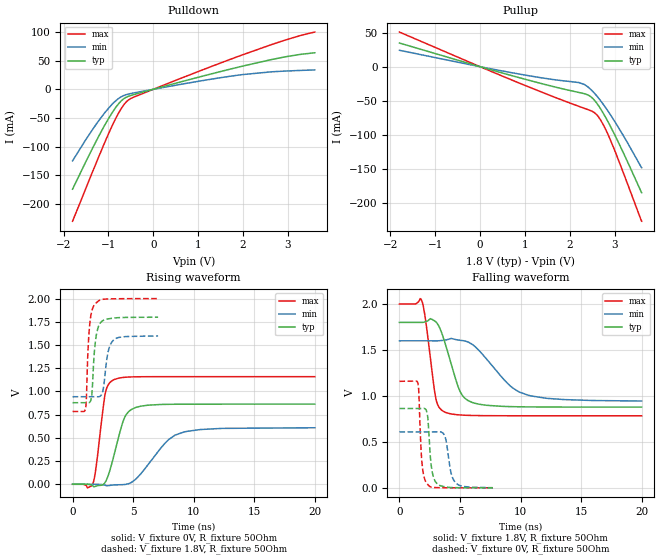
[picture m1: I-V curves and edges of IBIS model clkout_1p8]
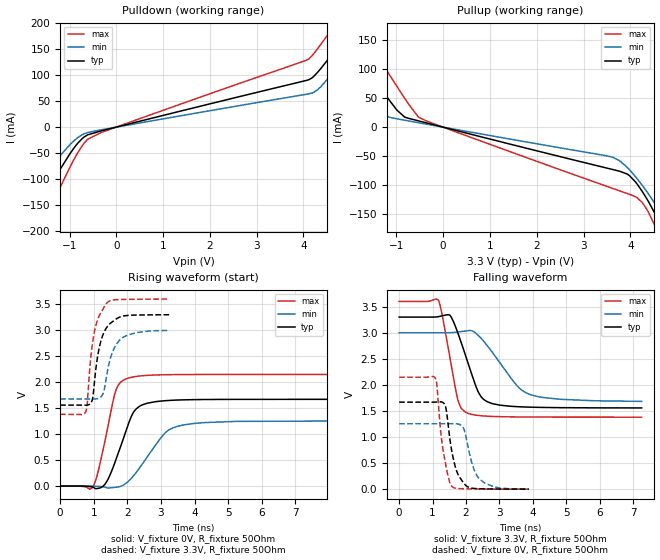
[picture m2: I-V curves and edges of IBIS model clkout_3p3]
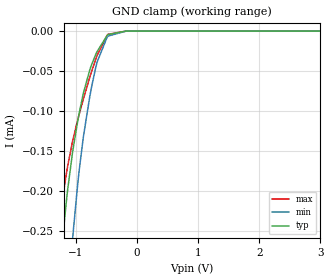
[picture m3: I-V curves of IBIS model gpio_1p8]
|Texas Instruments Incorporated
| TPS657095 Embedded Camera Module PMIC
| Marketing part#   Digital Voltage Range   Package-type   #pins
| TPS657095YFFR   3.7V-6V   DSBGA   16
| TPS657095YFFT   3.7V-6V   DSBGA   16
[IBIS Ver]   4.1
[File name]   tps657095.ibs
[File Rev]   1.0
[Date]   9/18/2015
[Source]
| Texas Instruments Incorporated.
| Analog-eLab Design Center, HPA
| 12500 TI Blvd
| Dallas, TX -75243
[Notes]   Revision History:
| Rev 1.0: 9/18/2015
| - Initial version of the model
| - Model generated from simulations in SPECTRE
| - Model matched to SPECTRE simulation
| - C_comp although listed in numerical order of value are
|   obtained from varying PVT conditions. For PVT conditions for
|   each specific value refer the buffer description under
|   respective [Model]. IBIS model user is responsible for using
|   appropriate C_comp to simulate for Signal Integrity.
|* EXCEPTION:   *
|* - For models clkout_*,there will be leakage in pullup/pulldown   *
|*   IV tables because of driver switch allignment.   *
[Disclaimer]
| This model is designed as an aid for customers of Texas Instruments.
| TI and its licensors and suppliers make no warranties, either expressed
| or implied, with respect to this  model, including the warranties of
| merchantability or fitness for a particular purpose. The model is
| provided solely on an "as is" basis. The entire risk as to its quality
| and performance is with the customer.
[Copyright]
(C) Copyright 2015 Texas Instruments Incorporated.All rights reserved.
|   TPS657095YFF
[Component]   TPS657095YFF
[Manufacturer]   TI
[Package]   |16 DSBGA - YFF package
|   typ   min   max
R_pkg   0.2   0.16   0.24
L_pkg   1.5nH   1.2nH   1.8nH
C_pkg   0.4pF   0.32pF   0.48pF
[Pin]  signal_name   model_name   R_pin   L_pin   C_pin
A1   VLDO2   nc   NA   NA   NA
A2   ISINK   nc   NA   NA   NA
A3   CLKOUT   clkout   NA   NA   NA
A4   X1   nc   NA   NA   NA
B1   GND   gnd   NA   NA   NA
B2   GPIO   gpio   NA   NA   NA
B3   SCL   sclk   NA   NA   NA
B4   X0   nc   NA   NA   NA
C1   VCC   power   NA   NA   NA
C2   LED_EN   leden   NA   NA   NA
C3   SDA   sda   NA   NA   NA
C4   AGND   gnd   NA   NA   NA
D1   VLDO1   nc   NA   NA   NA
D2   GPO   gpo   NA   NA   NA
D3   VCC   power   NA   NA   NA
D4   AVCC   power   NA   NA   NA
|   Model Selectors
[Model Selector] leden
leden_3p3   3.3V   digital Input
leden_1p8   1.8V   digital Input
leden_5   5V   digital Input
[Model Selector] gpio
gpio_3p3  3.3V   digital Input
gpio_1p8  1.8V   digital Input
[Model Selector] sclk
sclk_3p3   3.3V   digital Input
sclk_5   5V   digital Input
[Model Selector] gpo
gpo_3p3   3.3V   digital Output
gpo_1p8   1.8V   digital Output
[Model Selector] clkout
clkout_3p3   3.3V   digital Output
clkout_1p8   1.8V   digital Output
[Model Selector] sda
sda_3p3   3.3V   digital I/O_open_drain
sda_5   5V   digital I/O_open_drain
| Models and submodels in the file (13): clkout_1p8 (Output), clkout_3p3 (Output), gpio_1p8 (Input), gpio_3p3 (Input), gpo_1p8 (3-state), gpo_3p3 (3-state), leden_1p8 (Input), leden_3p3 (Input), leden_5 (Input), sclk_3p3 (Input), sclk_5 (Input), sda_3p3 (I/O_open_drain), sda_5 (I/O_open_drain)
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|   clkout_1p8 Model
[Model]   clkout_1p8
Model_type   Output
Polarity   Inverting
Vmeas = 0.9
Vref = 0
Cref = 2pF
Rref = 120
|   typ   min   max
|   (nom PVT)   (fast PVT)   (slow PVT)
C_comp   5.265e-13   4.178e-13   6.814e-13
| Where nom  PVT is Nominal Process, 1.8V, 27C
|   Fast PVT is Strong Process,  2V, -40C
|   Slow PVT is Weak Process,   1.6V, 125C
[Voltage Range]   1.8   1.6   2
|Junction Temperature
[Temperature Range]   27   125   -40
[Pullup Reference]   1.8   1.6   2
[Pulldown Reference]   0   0   0
[Power Clamp Reference]   1.8   1.6   2
[GND Clamp Reference]   0   0   0
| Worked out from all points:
|   slope of the pulldown table from 0 to 0.27 V, typ, clamps not added: 47.1 ohm
|   slope of the pullup table from 0 to 0.27 V, typ, clamps not added: 53.2 ohm
|   falling waveform, V_fixture 1.8V, R_fixture 50Ohm: 20-80 % time 1.29ns typ, 2.74ns min, 702ps max; typ from 1.8 V to 0.879 V
|   rising waveform, V_fixture 0V, R_fixture 50Ohm: 20-80 % time 1.08ns typ, 2.3ns min, 643ps max; typ from 0 V to 0.863 V
|   rising waveform, V_fixture 1.8V, R_fixture 50Ohm: 20-80 % time 332ps typ, 426ps min, 280ps max; typ from 0.879 V to 1.8 V
|   falling waveform, V_fixture 0V, R_fixture 50Ohm: 20-80 % time 321ps typ, 462ps min, 260ps max; typ from 0.863 V to 0 V
[Pulldown]
|   Voltage   I(typ)   I(min)   I(max)
-1.8V     -174.2mA   -124.8mA   -230.2mA
-1.344V   -101.2mA   -68.93mA   -142mA
-988.8mV  -49.85mA   -32.18mA   -75.97mA
-876mV    -35.94mA   -22.84mA   -56.86mA
-755.2mV  -23.5mA    -15.02mA   -38.84mA
-656mV    -16.31mA   -10.81mA   -26.84mA
-558mV    -12.26mA   -8.351mA   -18.8mA
-462mV    -9.855mA   -6.717mA   -14.54mA
450mV     9.562mA    6.42mA     14.09mA
1.976V    40.2mA     25.57mA    59.79mA
2.928V    56.47mA    31.79mA    85.55mA
3.6V      63.73mA    33.82mA    99.91mA
[Pullup]
|   Voltage   I(typ)   I(min)   I(max)
-1.8V     34.79mA    24.14mA    50.93mA
736mV     -13.69mA   -9.206mA   -20.39mA
1.525V    -27.44mA   -17.89mA   -41.36mA
2.203V    -37.88mA   -23.35mA   -58.35mA
2.408V    -41.68mA   -30.01mA   -63.21mA
2.555V    -49.87mA   -39.52mA   -67.97mA
2.619V    -55.38mA   -44.49mA   -72.17mA
2.696V    -63.15mA   -51.01mA   -79.64mA
2.783V    -72.82mA   -58.83mA   -90.19mA
2.892V    -86.14mA   -69.41mA   -105.9mA
3.178V    -124.5mA   -99.75mA   -153.4mA
3.6V      -185.1mA   -148.5mA   -227.2mA
[Ramp]
R_load = 50
|   typ   min   max
dV/dt_r   0.517849/1.07589e-09   0.365218/2.28825e-09   0.695442/6.41697e-10
dV/dt_f   0.552848/1.29077e-09   0.393134/2.70964e-09   0.729524/7.00502e-10
[Falling Waveform]
V_fixture = 1.8V
V_fixture_min = 1.6V
V_fixture_max = 2V
R_fixture = 50Ohm
|   Time   V(typ)   V(min)   V(max)
0s        1.8V       1.6V       2V
1.838ns   1.8V       1.6V       2.039V
2.117ns   1.806V     1.6V       1.864V
3ns       1.807V     1.6V       977.3mV
3.722ns   1.594V     1.607V     826mV
4.981ns   1.057V     1.606V     793.4mV
6.099ns   925.5mV    1.553V     787.2mV
9.129ns   884.1mV    1.112V     784.4mV
10.67ns   880.7mV    1.006V     784.2mV
20ns      878.6mV    944.8mV    784.1mV
[Rising Waveform]
V_fixture = 0V
V_fixture_min = 0V
V_fixture_max = 0V
R_fixture = 50Ohm
|   Time   V(typ)   V(min)   V(max)
0s        177.8pV    11.09nV    15.52pV
1.676ns   -17.43mV   36.1uV     3.913mV
1.942ns   -19.31mV   100.4uV    182.9mV
2.7ns     21.99mV    -10.59mV   978.1mV
3.433ns   318.7mV    -7.003mV   1.128V
4.317ns   724mV      -2.543mV   1.152V
5.332ns   831.5mV    69.27mV    1.158V
7.935ns   861.1mV    481.4mV    1.159V
9.249ns   862.4mV    564.7mV    1.159V
20ns      863.1mV    608.7mV    1.159V
[Rising Waveform]
V_fixture = 1.8V
V_fixture_min = 1.6V
V_fixture_max = 2V
R_fixture = 50Ohm
|   Time   V(typ)   V(min)   V(max)
0s        878.5mV    943mV      784.1mV
1.068ns   878.6mV    943mV      812.4mV
1.379ns   879.9mV    943.1mV    1.668V
1.591ns   962.3mV    943.1mV    1.866V
1.807ns   1.437V     943.1mV    1.934V
2.08ns    1.676V     942.4mV    1.968V
2.471ns   1.76V      989.7mV    1.992V
2.912ns   1.781V     1.414V     1.996V
3.32ns    1.789V     1.545V     1.997V
7.062ns   1.8V       1.598V     2V
[Falling Waveform]
V_fixture = 0V
V_fixture_min = 0V
V_fixture_max = 0V
R_fixture = 50Ohm
|   Time   V(typ)   V(min)   V(max)
0s        863.1mV    608.9mV    1.159V
1.517ns   863.1mV    608.9mV    1.142V
1.911ns   863.9mV    608.9mV    207.7mV
2.406ns   651mV      608.9mV    26.5mV
2.707ns   173.3mV    608.9mV    5.756mV
3.171ns   37.26mV    610.1mV    2.202mV
3.746ns   11.98mV    566.6mV    1.191mV
4.268ns   3.672mV    159.3mV    799.8uV
4.669ns   2.019mV    51.11mV    617.3uV
7.722ns   418.2uV    1.702mV    156.5uV
|   clkout_3p3 Model
[Model]   clkout_3p3
Model_type   Output
Polarity   Inverting
Vmeas = 1.65
Vref = 0
Cref = 2pF
Rref = 100
|   typ   min   max
|   (nom PVT)   (fast PVT)   (slow PVT)
C_comp   5.420e-13   4.378e-13   6.661e-13
| Where nom  PVT is Nominal Process, 3.3V, 27C
|   Fast PVT is Strong Process,  3.6V, -40C
|   Slow PVT is Weak Process,   3V, 125C
[Voltage Range]   3.3   3   3.6
|Junction Temperature
[Temperature Range]   27   125   -40
[Pullup Reference]   3.3   3   3.6
[Pulldown Reference]   0   0   0
[Power Clamp Reference]   3.3   3   3.6
[GND Clamp Reference]   0   0   0
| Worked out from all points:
|   slope of the pulldown table from 0 to 0.495 V, typ, clamps not added: 44.5 ohm
|   slope of the pullup table from 0 to 0.495 V, typ, clamps not added: 48.6 ohm
|   falling waveform, V_fixture 3.3V, R_fixture 50Ohm: 20-80 % time 558ps typ, 928ps min, 376ps max; typ from 3.3 V to 1.56 V
|   rising waveform, V_fixture 0V, R_fixture 50Ohm: 20-80 % time 555ps typ, 845ps min, 419ps max; typ from 0 V to 1.67 V
|   rising waveform, V_fixture 3.3V, R_fixture 50Ohm: 20-80 % time 292ps typ, 338ps min, 259ps max; typ from 1.56 V to 3.3 V
|   falling waveform, V_fixture 0V, R_fixture 50Ohm: 20-80 % time 280ps typ, 335ps min, 241ps max; typ from 1.67 V to 0.001 V
[Pulldown]
|   Voltage   I(typ)   I(min)   I(max)
-3.3V     -558.5mA   -389.9mA   -709mA
-2.314V   -260.4mA   -194.9mA   -340.7mA
-1.805V   -176.8mA   -127.5mA   -232.8mA
-1.449V   -119mA     -82.82mA   -163.3mA
-980.1mV  -49.67mA   -32.59mA   -75.17mA
-683.1mV  -18.65mA   -12.65mA   -30.31mA
-330mV    -7.359mA   -5.21mA    -10.55mA
4.179V    94.46mA    65.46mA    136.9mA
4.372V    112.7mA    77.68mA    159.2mA
4.864V    169mA      128.4mA    220.9mA
4.971V    181.5mA    140.1mA    234.5mA
6.6V      374.4mA    321.3mA    441.6mA
[Pullup]
|   Voltage   I(typ)   I(min)   I(max)
-3.3V     300mA      240.5mA    366.6mA
-1.884V   131.4mA    82.24mA    184.4mA
-1.64V    102.7mA    56.08mA    153.2mA
-1.152V   46.66mA    17.03mA    91.05mA
-821.7mV  17.31mA    11.96mA    49.8mA
-528mV    10.84mA    7.658mA    17.23mA
3.634V    -73.48mA   -52.44mA   -106.2mA
3.933V    -81.14mA   -69.5mA    -114.7mA
4.115V    -95.23mA   -86.14mA   -120.5mA
4.75V     -182.5mA   -159.2mA   -207.8mA
4.932V    -211.2mA   -182.3mA   -241.7mA
6.6V      -614.3mA   -519mA     -687.7mA
[Ramp]
R_load = 50
|   typ   min   max
dV/dt_r   1.00131/5.5446e-10   0.752779/8.44337e-10   1.28864/4.18949e-10
dV/dt_f   1.04549/5.5682e-10   0.793395/9.3373e-10   1.33129/3.74911e-10
[Falling Waveform]
V_fixture = 3.3V
V_fixture_min = 3V
V_fixture_max = 3.6V
R_fixture = 50Ohm
|   Time   V(typ)   V(min)   V(max)
0s        3.3V       3V         3.6V
1.179ns   3.309V     3V         3.619V
1.517ns   3.336V     3.001V     2.527V
1.759ns   2.989V     3.015V     1.708V
2.072ns   2.393V     3.04V      1.452V
2.361ns   1.869V     2.952V     1.414V
2.556ns   1.708V     2.815V     1.403V
3.482ns   1.584V     2.016V     1.386V
3.836ns   1.575V     1.835V     1.384V
7.249ns   1.558V     1.684V     1.381V
[Rising Waveform]
V_fixture = 0V
V_fixture_min = 0V
V_fixture_max = 0V
R_fixture = 50Ohm
|   Time   V(typ)   V(min)   V(max)
0s        206.7pV    8.889nV    24.3pV
976.7ps   -21.55mV   -836.2uV   -11.96mV
1.338ns   38.12mV    -21.03mV   879.1mV
1.644ns   478.2mV    -24.77mV   1.812V
2.014ns   1.16V      80.09mV    2.073V
2.213ns   1.447V     219.7mV    2.104V
2.437ns   1.559V     415.1mV    2.122V
3.119ns   1.642V     1.019V     2.142V
3.641ns   1.658V     1.172V     2.145V
10ns      1.669V     1.255V     2.148V
[Rising Waveform]
V_fixture = 3.3V
V_fixture_min = 3V
V_fixture_max = 3.6V
R_fixture = 50Ohm
|   Time   V(typ)   V(min)   V(max)
0s        1.557V     1.676V     1.381V
765.5ps   1.555V     1.676V     1.432V
922.5ps   1.604V     1.676V     2.533V
1.004ns   1.889V     1.675V     2.914V
1.15ns    2.617V     1.69V      3.258V
1.288ns   2.933V     1.792V     3.419V
1.376ns   3.043V     2.089V     3.511V
1.562ns   3.165V     2.587V     3.578V
1.842ns   3.267V     2.847V     3.59V
3.252ns   3.297V     2.994V     3.598V
[Falling Waveform]
V_fixture = 0V
V_fixture_min = 0V
V_fixture_max = 0V
R_fixture = 50Ohm
|   Time   V(typ)   V(min)   V(max)
0s        1.669V     1.255V     2.148V
1.085ns   1.67V      1.255V     2.124V
1.131ns   1.672V     1.255V     1.975V
1.256ns   1.674V     1.255V     1.024V
1.387ns   1.587V     1.255V     492.1mV
1.612ns   607.6mV    1.258V     35.74mV
1.916ns   131.2mV    1.182V     7.995mV
2.235ns   15.05mV    379.2mV    4.36mV
2.41ns    8.363mV    191.6mV    3.382mV
3.874ns   1.498mV    3.583mV    880.5uV
|   gpio_1p8 Model
[Model]   gpio_1p8
Model_type   Input
Vinl = 0.4
Vinh = 1.1
|   typ   min   max
|   (nom PVT)   (fast PVT)   (slow PVT)
C_comp   5.874e-13   5.404e-13   6.639e-13
| Where nom  PVT is Nominal Process, 1.8V, 27C
|   Fast PVT is Strong Process,  2V, -40C
|   Slow PVT is Weak Process,   1.6V, 125C
[Voltage Range]   1.8   1.6   2
|Junction Temperature
[Temperature Range]   27   125   -40
[Power Clamp Reference]   1.8   1.6   2
[GND Clamp Reference]   0   0   0
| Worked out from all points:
|   GND clamp passes 1 mA (typ) near -1.75 V on its own axis
[GND Clamp]
|   Voltage   I(typ)   I(min)   I(max)
-1.8V     -1.081mA   -1.499mA   -1.058mA
-1.309V   -352.2uA   -562.9uA   -269.4uA
-1.273V   -313.2uA   -510.8uA   -242.1uA
-1.206V   -250.5uA   -422.7uA   -202.1uA
-1.136V   -197.8uA   -340.6uA   -168.7uA
-1.05V    -148.4uA   -254.6uA   -135.6uA
-881.6mV  -78.21uA   -133.3uA   -85.55uA
-774.4mV  -48.38uA   -81.59uA   -57.66uA
-657mV    -25.82uA   -39.18uA   -30.81uA
-474mV    -4.28uA    -6.197uA   -3.987uA
-180mV    0A         -40.11nA   0A
3.6V      0A         0A         0A
[POWER Clamp]
|   Voltage   I(typ)   I(min)   I(max)
-1.8V     0A         0A         0A
0V        0A         0A         0A
3.6V      0A         0A         0A
